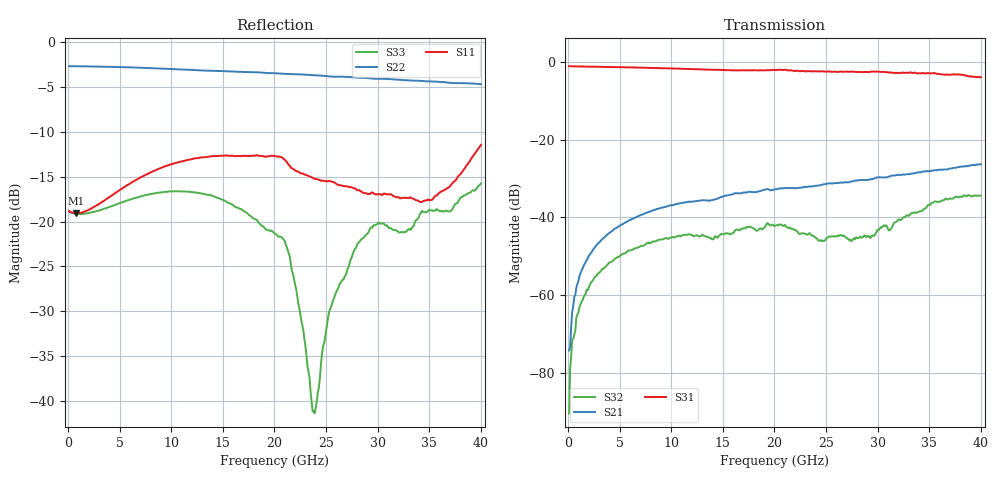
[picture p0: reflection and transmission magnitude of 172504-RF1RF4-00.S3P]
!  3-Port S-parameters saved by WinCal
! VAR MeasName=S-Parameters (CALIBRATED_DATA) read from VNA (N5245A)
! VAR MeasDate=2017-3-15 11:11:18
! VAR NAME=172504-RF1RF4-00
! VAR FILENAME=172504-RF1RF4-00.S3P
! VAR DATE=2017-3-15 11:11:18
! VAR PHYS_PORTS=1,2,3
# Hz S DB R 50
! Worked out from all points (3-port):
!   400 points, 100 MHz to 40 GHz, reference 50 ohm
!   strongest paths, dB at 100 MHz, 10.1 GHz, 20.1 GHz, 30.1 GHz, 40 GHz:
!     S31: -1.1, -1.7, -2.1, -2.5, -3.9
!     S21: -74.2, -36.9, -32.8, -29.7, -26.3
!     S32: -90.4, -45.1, -42.1, -43.3, -34.4
!   lowest |S11| = -19.1 dB at 800 MHz (marker M1), VSWR 1.25, Z = 61.9 - j3.66 ohm
!   |S11| at or under -10 dB: start of sweep to end of sweep
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1e8  -18.83 -2.6  -76.70 71.7  -1.10 -0.7
     -74.24 94.5  -2.66 179.8  -91.70 -19.2
     -1.10 -0.7  -90.42 18.0  -18.85 -2.3
3e8  -18.97 -6.5  -66.12 104.7  -1.12 -2.0
     -68.18 106.8  -2.66 179.3  -73.61 134.5
     -1.12 -2.0  -75.70 92.7  -19.00 -5.7
8e8  -19.07 -15.2  -58.18 91.8  -1.16 -5.1
     -58.09 91.6  -2.67 178.3  -65.93 100.3
     -1.16 -5.1  -65.82 101.7  -19.13 -13.2
5.7e9  -15.93 -76.5  -41.14 61.8  -1.38 -33.7
       -41.11 62.5  -2.78 168.1  -48.69 51.8
       -1.39 -33.7  -48.84 51.2  -17.64 -73.3
2.01e10  -12.69 -154.8  -32.51 -2.9  -2.08 -113.9
         -32.76 -1.7  -3.45 137.8  -42.30 -39.8
         -2.10 -113.6  -42.11 -43.9  -21.39 -174.9
2.15e10  -13.81 -164.3  -32.39 -11.4  -2.24 -123.7
         -32.49 -8.8  -3.54 134.6  -42.48 -55.4
         -2.20 -122.9  -42.63 -57.0  -24.00 156.4
2.39e10  -15.23 -165.3  -31.95 -19.1  -2.46 -136.6
         -31.92 -16.0  -3.67 128.7  -44.94 -67.5
         -2.41 -136.2  -45.03 -69.9  -41.39 39.4
2.53e10  -15.45 -166.6  -31.35 -24.6  -2.58 -144.6
         -31.23 -22.8  -3.78 125.3  -44.71 -57.5
         -2.46 -144.8  -44.88 -59.4  -30.07 -26.7
2.81e10  -16.49 -175.0  -30.60 -37.3  -2.77 -161.6
         -30.54 -35.5  -3.95 118.2  -45.76 -62.0
         -2.58 -161.3  -45.40 -60.2  -22.40 -48.5
4e10  -11.44 34.2  -26.16 -108.6  -3.95 116.6
      -26.33 -108.9  -4.67 82.5  -34.87 -134.5
      -3.92 115.9  -34.43 -140.1  -15.75 -49.5
